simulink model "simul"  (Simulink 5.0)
settings: Solver=ode4  StartTime=0.0  StopTime=cas_simulacie  FixedStep=krok  RelTol=1e-3
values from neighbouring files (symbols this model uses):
  D = uicontrol(gcf,   'Style','edit',   'ForegroundColor','black',   'BackgroundColor',[1 1 1],   'String',num2str(D),   'Position',[100 105 80 20],   'CallBack',['D=str2num(get(D,''String''));'])    [id_system.m]    (also in param.m = D1; param2.m = D2)
  dolna_hranica_akcnej_veliciny = uicontrol(gcf,   'Style','edit',   'ForegroundColor','black',   'BackgroundColor',[1 1 1],   'String', num2str(dolna_hranica_akcnej_veliciny),   'Position',[195 80 80 20],   'CallBack',['dolna_hranica_akcnej_veliciny=str2num(get(dolna_hranica_akcnej_veliciny,''String''));'])    [simul_param.m]
  horna_hranica_akcnej_veliciny = uicontrol(gcf,   'Style','edit',   'ForegroundColor','black',   'BackgroundColor',[1 1 1],   'String',num2str(horna_hranica_akcnej_veliciny),   'Position',[195 50 80 20],   'CallBack',['horna_hranica_akcnej_veliciny=str2num(get(horna_hranica_akcnej_veliciny,''String''));'])    [simul_param.m]
  presnost_riadenia = uicontrol(gcf,   'Style','edit',   'ForegroundColor','black',   'BackgroundColor',[1 1 1],   'String',num2str(presnost_riadenia),   'Position',[125 110 80 20],   'CallBack',['presnost_riadenia=str2num(get(presnost_riadenia,''String''));'])    [simul_param.m]
  T = uicontrol(gcf,   'Style','edit',   'ForegroundColor','black',   'BackgroundColor',[1 1 1],   'String',num2str(T),   'Position',[100 80 80 20],    'CallBack',['T=str2num(get(T,''String''));'])    [id_system.m]    (also in param.m = T1; param2.m = T2)
  t_d = T_D    [pid_param.m]    (also in pi_param.m = 0; p_param.m = 0)
  t_i = T_I    [pid_param.m]    (also in pi_param.m; p_param.m = 10000000000)
  u_0 = uicontrol(gcf,   'Style','edit',   'ForegroundColor','black',   'BackgroundColor',[1 1 1],   'String',num2str(u_0),   'Position',[100 230 80 20],   'CallBack',['u_0=str2num(get(u_0,''String''));'])    [id_system.m]    (also in sus1.m = uicontrol(gcf,   'Style','edit',   'ForegroundColor','black'; sus2.m = uicontrol(gcf,   'Style','edit',   'ForegroundColor','black')
  y_0 = uicontrol(gcf,   'Style','edit',   'ForegroundColor','black',   'BackgroundColor',[1 1 1],   'String', num2str(y_0),   'Position',[100 180 80 20],   'CallBack',['y_0=str2num(get(y_0,''String''));'])    [id_system.m]    (also in sus1.m = uicontrol(gcf,   'Style','edit',   'ForegroundColor','black'; sus2.m = uicontrol(gcf,   'Style','edit',   'ForegroundColor','black')
  Z = uicontrol(gcf,   'Style','edit',   'ForegroundColor','black',   'BackgroundColor',[1 1 1],   'String',num2str(Z) ,   'Position',[100 130 80 18],   'CallBack',['Z=str2num(get(Z,''String''));'])    [id_system.m]    (also in param.m = Z1; param2.m = Z2)
  z_r = Z_R    [pid_param.m]    (also in pi_param.m; p_param.m)
  ziadana_hodnota = uicontrol(gcf,   'Style','edit',   'ForegroundColor','black',   'BackgroundColor',[1 1 1],   'String',num2str(ziadana_hodnota),   'Position',[125 140 80 20],   'CallBack',['ziadana_hodnota=str2num(get(ziadana_hodnota,''String''));'])    [simul_param.m]
libraries: simulink_extras x1

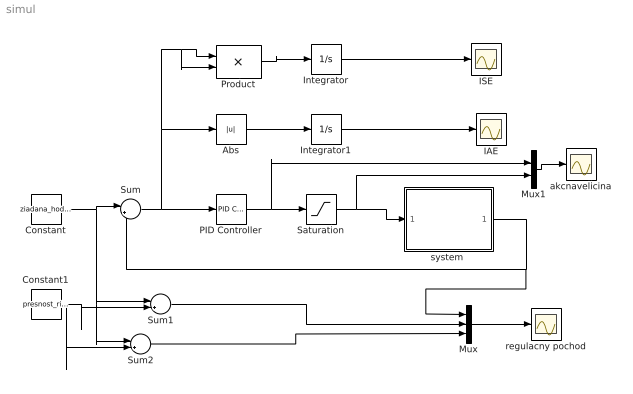
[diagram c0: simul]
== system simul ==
  Abs : Abs
  Constant : Constant  Value=ziadana_hodnota
  Constant1 : Constant  Value=presnost_riadenia
  IAE : Scope
  ISE : Scope
  Integrator : Integrator
  Integrator1 : Integrator
  Mux : Mux  Inputs=3
  Mux1 : Mux  Inputs=2
  PID Controller : simulink_extras/Additional Linear/PID Controller  P=z_r  I=z_r/t_i  D=z_r*t_d
  Product : Product
  Saturation : Saturate  UpperLimit=horna_hranica_akcnej_veliciny  LowerLimit=dolna_hranica_akcnej_veliciny
  Sum : Sum  Inputs=|+-
  Sum1 : Sum  Inputs=|++
  Sum2 : Sum  Inputs=|+-
  akcnavelicina : Scope
  regulacny pochod : Scope
  "system " : Subsystem
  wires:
  Constant/1 -> Sum/1, Sum2/1, Sum1/1
  Sum/1 -> Abs/1, Product/2, Product/1, PID Controller/1
  PID Controller/1 -> Saturation/1, Mux1/1
  Saturation/1 -> "system "/1(In1), Mux1/2
  Abs/1 -> Integrator1/1
  Integrator/1 -> ISE/1
  Integrator1/1 -> IAE/1
  Constant1/1 -> Sum1/2, Sum2/2
  Mux/1 -> regulacny pochod/1
  "system "/1(Out1) -> Mux/1, Sum/2
  Sum2/1 -> Mux/3
  Sum1/1 -> Mux/2
  Product/1 -> Integrator/1
  Mux1/1 -> akcnavelicina/1

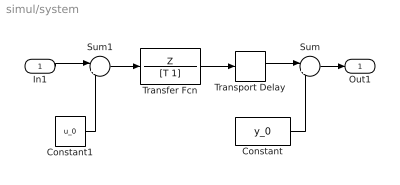
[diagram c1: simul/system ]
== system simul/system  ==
  In1 : Inport
  Constant : Constant  Value=y_0
  Constant1 : Constant  Value=u_0
  Sum : Sum  Inputs=|++
  Sum1 : Sum  Inputs=|+-
  Transfer Fcn : TransferFcn  Numerator=Z  Denominator=[T 1]
  Transport Delay : TransportDelay  DelayTime=D
  Out1 : Outport
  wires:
  Transfer Fcn/1 -> Transport Delay/1
  Transport Delay/1 -> Sum/1
  Constant/1 -> Sum/2
  Sum1/1 -> Transfer Fcn/1
  Constant1/1 -> Sum1/2
  In1/1 -> Sum1/1
  Sum/1 -> Out1/1
